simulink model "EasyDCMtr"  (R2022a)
settings: Solver=VariableStepAuto  StartTime=0.0  StopTime=10.0  RelTol=1e-3
libraries: simulink x1

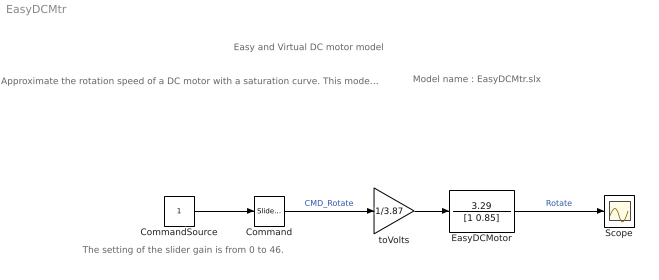
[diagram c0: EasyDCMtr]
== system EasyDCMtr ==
  note: The setting of the slider gain is from 0 to 46.
  note: Approximate the rotation speed of a DC motor with a saturation curve. This model specifies a rotation speed command (0 to 46rad/s) with a slider gain.
  note: Model name : EasyDCMtr.slx
  note: Easy and Virtual DC motor model
  Command : simulink/Math Operations/Slider Gain  gain=46.0  low=0  high=46
  CommandSource : Constant
  EasyDCMotor : TransferFcn  Numerator=3.29  Denominator=[1 0.85]
  Scope : Scope
  toVolts : Gain  Gain=1/3.87
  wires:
  toVolts/1 -> EasyDCMotor/1
  Command/1 -> toVolts/1  "CMD_Rotate"
  CommandSource/1 -> Command/1
  EasyDCMotor/1 -> Scope/1  "Rotate"
